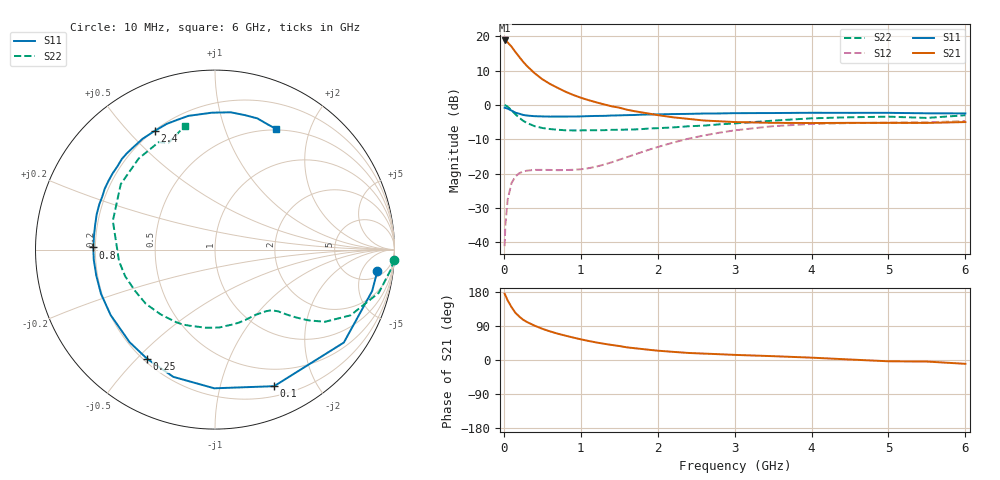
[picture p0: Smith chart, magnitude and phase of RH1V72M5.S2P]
! SIEMENS Small Signal Semiconductors
! BFR106
! Si NPN RF Bipolar Junction Transistor in SOT23
! VCE = 1.75 V  IC = 2.5 mA
! Common Emitter S-Parameters:  August  1996
# GHz  S  MA  R  50
!  f  S11  S21  S12  S22
! GHz  MAG  ANG  MAG  ANG  MAG  ANG  MAG  ANG
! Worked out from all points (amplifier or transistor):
!   36 points, 10 MHz to 6 GHz, reference 50 ohm
!   highest |S21| = 18.8 dB at 10 MHz (marker M1)
!   |S21| within 3 dB of that: start of sweep to 138.9 MHz
!   unconditionally stable (mu >= 1): 738.3 MHz to 2.293 GHz; 3.258 GHz to end of sweep
!   at 250 MHz: K = 0.36, MSG = 16.0 dB, |S12| = -19.4 dB
!   at 1.4 GHz: K = 1.27, MAG = 5.0 dB, |S12| = -16.7 dB
!   at 6 GHz: K = 1.02, MAG = -1.1 dB, |S12| = -4.7 dB
!   S11 on the Smith chart (normalised r, x): 10 MHz: 7, -10; 100 MHz: 0.30, -1.48; 250 MHz: 0.21, -0.54; 800 MHz: 0.19, +0.01; 2.4 GHz: 0.20, +0.59; 6 GHz: 0.49, +1.51
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0.01  0.9124 -7.6  8.692 174.7  0.0088 86.5  0.9967 -3.2
0.02  0.9054 -14.8  8.645 170.8  0.0178 83.4  0.9877 -6.2
0.05  0.8851 -35.8  8.127 157.1  0.0422 70.5  0.9436 -14.8
0.1  0.8292 -66.6  7.064 139.5  0.073 55.6  0.8388 -25.9
0.15  0.7728 -90.3  5.916 124.6  0.0909 44.2  0.7326 -33.3
0.2  0.7461 -108.1  5.01 114.8  0.1015 37.5  0.6535 -37.1
0.25  0.7166 -121.8  4.263 106.3  0.1075 32.2  0.5896 -39.9
0.3  0.7018 -132.7  3.698 100.3  0.1106 29.5  0.5471 -41.8
0.4  0.6863 -147.9  2.901 90.6  0.1135 25.9  0.4915 -44.4
0.5  0.6813 -158.8  2.368 82.4  0.1136 24.7  0.4622 -47.0
0.6  0.6771 -167.7  2.025 75.5  0.1133 25.4  0.446 -50.3
0.8  0.6781 179.0  1.562 64.3  0.1128 30.0  0.428 -58.0
1.1  0.688 163.3  1.176 50.3  0.12 41.7  0.428 -71.6
1.6  0.7112 143.2  0.853 33.4  0.1738 57.2  0.4383 -97.2
2.2  0.7374 123.2  0.661 21.5  0.2835 56.5  0.4713 -130.2
2.4  0.7418 117.0  0.627 18.6  0.3231 53.5  0.4895 -141.9
3  0.7597 101.2  0.564 13.5  0.4272 41.3  0.5386 -173.1
3.5  0.763 91.3  0.549 10.1  0.4914 30.4  0.5912 164.3
4.5  0.7675 77.4  0.549 1.3  0.5448 11.2  0.662 130.0
5  0.7682 72.1  0.549 -3.4  0.5535 3.9  0.6756 117.7
5.5  0.7563 66.8  0.548 -4.1  0.5601 0.6  0.6478 113.6
6  0.7536 63.3  0.564 -10.1  0.5816 -6.8  0.7087 103.8
